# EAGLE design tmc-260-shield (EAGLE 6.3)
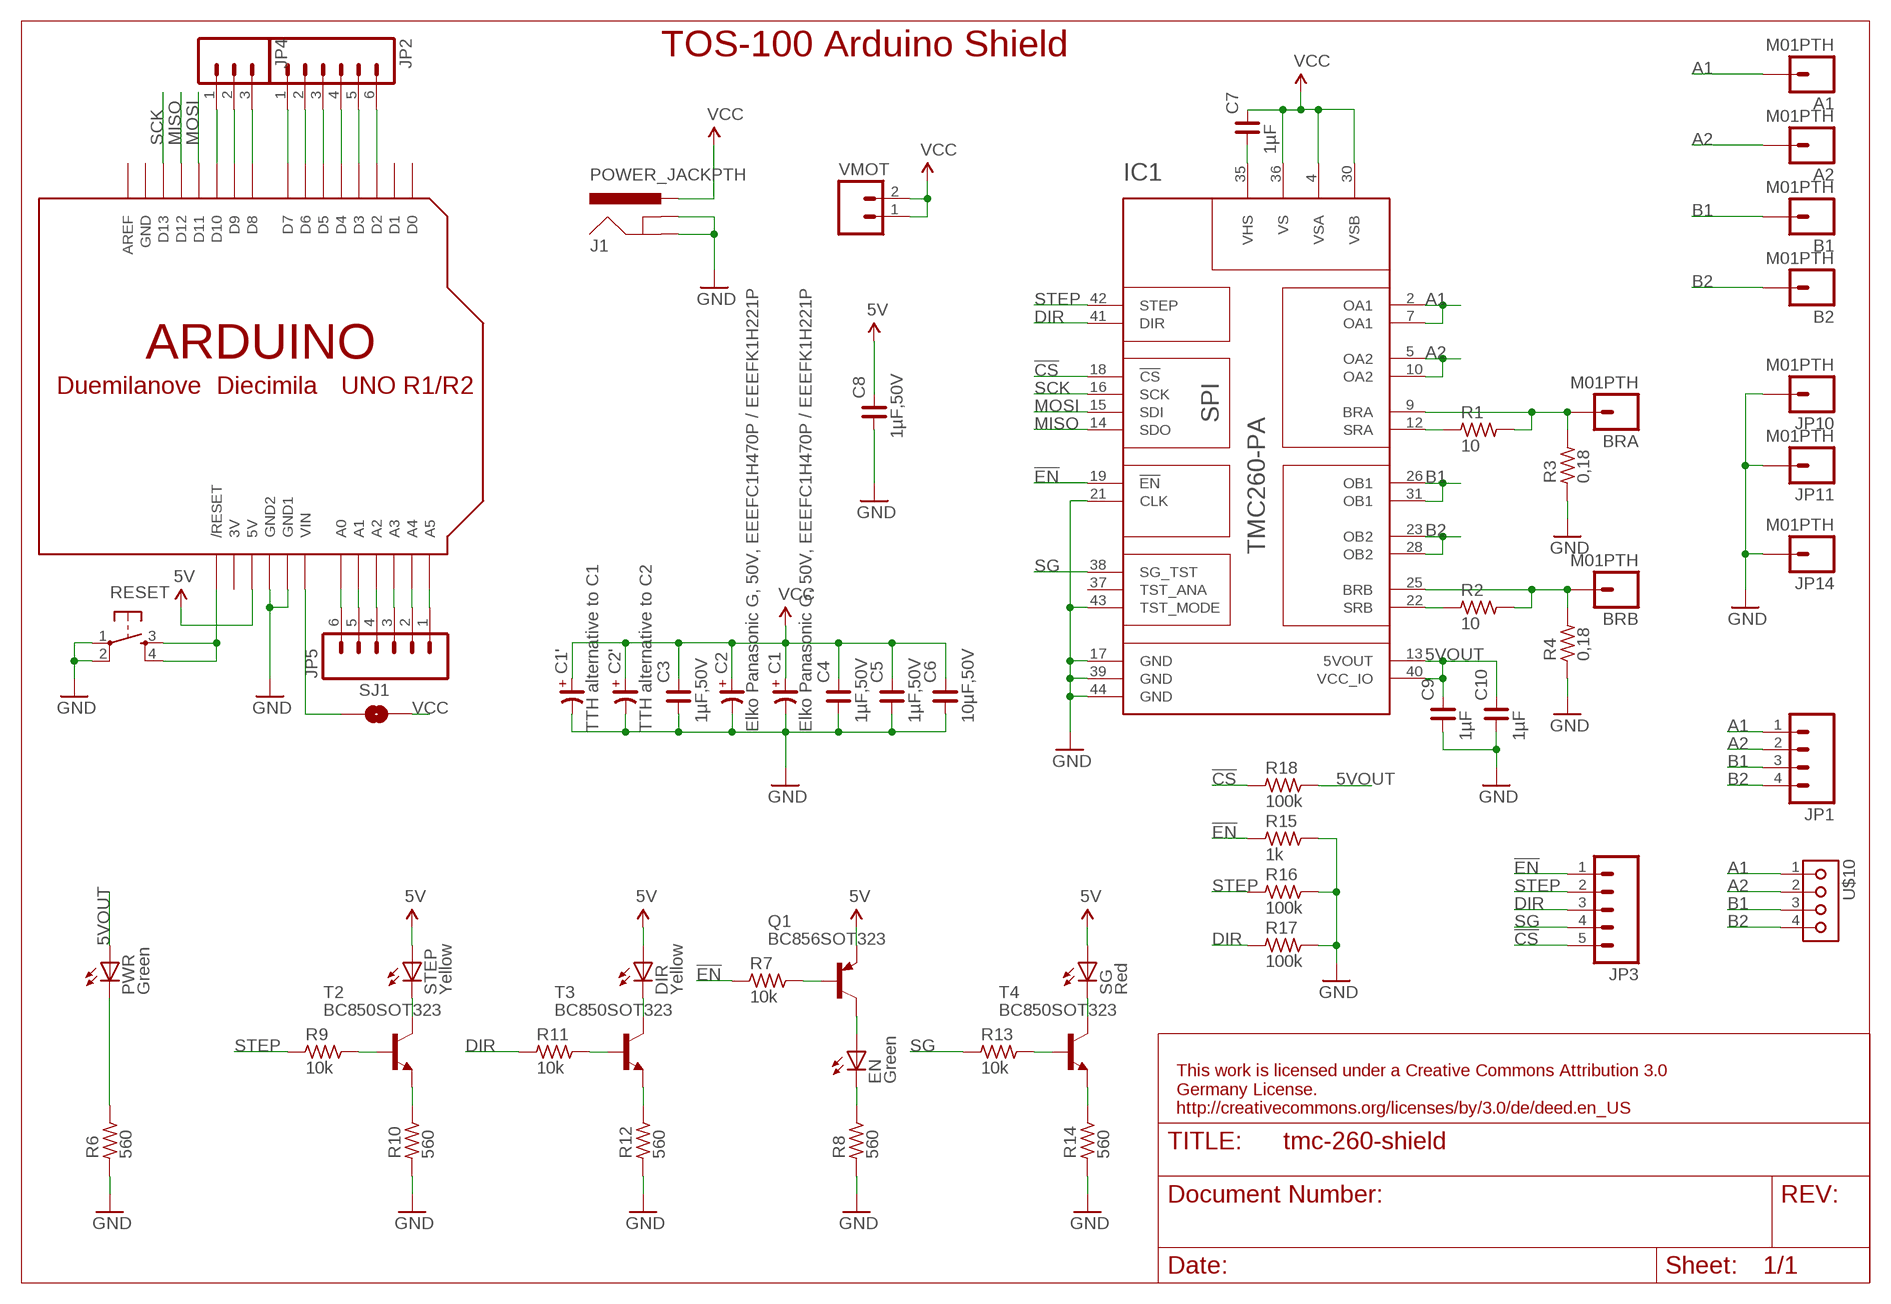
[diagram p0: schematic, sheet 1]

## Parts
A1  M01PTH  [1X01]
A2  M01PTH  [1X01]
B1  M01PTH  [1X01]
B2  M01PTH  [1X01]
BRA  M01PTH  [1X01]
BRB  M01PTH  [1X01]
C1  Elko Panasonic G, 50V, EEEFC1H470P / EEEFK1H221P  CP_SV-G  [CSV-G]
C1'  TTH alternative to C1  CP_E-035X100  [CE-035X100]
C2  Elko Panasonic G, 50V, EEEFC1H470P / EEEFK1H221P  CP_SV-G  [CSV-G]
C2'  TTH alternative to C2  CP_E-035X100  [CE-035X100]
C3  1µF,50V  C_0603  [C0603]
C4  1µF,50V  C_0603  [C0603]
C5  1µF,50V  C_0603  [C0603]
C6  10µF,50V  C_1206  [C1206]
C7  1µF  C_0603  [C0603]
C8  1µF,50V  C_0603  [C0603]
C9  1µF  C_0603  [C0603]
C10  1µF  C_0603  [C0603]
DIR  Yellow  LEDMICRO-SIDELED  [MICRO-SIDELED]
EN  Green  LEDMICRO-SIDELED  [MICRO-SIDELED]
IC1  TMC260-PA  [PQFP44_WITH_PADS]
J1  POWER_JACKPTH  [POWER_JACK_PTH]
JP1  M04SCREW  [SCREWTERMINAL-3.5MM-4]
JP2  M06SIP  [1X06]
JP3  M05PTH  [1X05]
JP4  M03PTH  [1X03]
JP5  M06SIP  [1X06]
JP10  M01PTH  [1X01]
JP11  M01PTH  [1X01]
JP14  M01PTH  [1X01]
PWR  Green  LEDMICRO-SIDELED  [MICRO-SIDELED]
Q1  BC856SOT323  BC858SOT323  [SOT323-BEC]
R1  10  R_0603  [R0603]
R2  10  R_0603  [R0603]
R3  0,18  R_2512  [R2512]
R4  0,18  R_2512  [R2512]
R6  560  R_0603  [R0603]
R7  10k  R_0603  [R0603]
R8  560  R_0603  [R0603]
R9  10k  R_0603  [R0603]
R10  560  R_0603  [R0603]
R11  10k  R_0603  [R0603]
R12  560  R_0603  [R0603]
R13  10k  R_0603  [R0603]
R14  560  R_0603  [R0603]
R15  1k  R_0603  [R0603]
R16  100k  R_0603  [R0603]
R17  100k  R_0603  [R0603]
R18  100k  R_0603  [R0603]
RESET  TAC_SWITCHSMD  [TACTILE_SWITCH_SMD]
SG  Red  LEDMICRO-SIDELED  [MICRO-SIDELED]
SJ1  SOLDERJUMPERNO  [SJ_2S-NO]
STEP  Yellow  LEDMICRO-SIDELED  [MICRO-SIDELED]
T2  BC850SOT323  [SOT323-BEC]
T3  BC850SOT323  [SOT323-BEC]
T4  BC850SOT323  [SOT323-BEC]
U$1  ARDUINOUNO  [ARDUINO]
U$10  KK4H  [KK-H-4]
VMOT  M021X02_NO_SILK  [1X02_NO_SILK]

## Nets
5V: C8.2 DIR.A Q1.E SG.A STEP.A U$1.5V
5VOUT: C9.2 C10.2 IC1.13(5VOUT) IC1.40(VCC_IO) PWR.A R18.2
!CS: IC1.18(!CS) JP3.5 R18.1
!EN: IC1.19(!EN) JP3.1 R7.1 R15.1
A1: A1.1 IC1.2(OA1) IC1.7(OA1) JP1.1 U$10.1
A2: A2.1 IC1.5(OA2) IC1.10(OA2) JP1.2 U$10.2
B1: B1.1 IC1.26(OB1) IC1.31(OB1) JP1.3 U$10.3
B2: B2.1 IC1.23(OB2) IC1.28(OB2) JP1.4 U$10.4
DIR: IC1.41(DIR) JP3.3 R11.1 R17.1
GND: C1'.- C1.- C2'.- C2.- C3.1 C4.1 C5.1 C6.1 C8.1 C9.1 C10.1 IC1.17(GND) IC1.21(CLK) IC1.39(GND) IC1.43(TST_MODE) IC1.44(GND) J1.GND J1.GNDBREAK JP10.1 JP11.1 JP14.1 R3.1 R4.1 R6.1 R8.1 R10.1 R12.1 R14.1 R15.2 R16.2 R17.2 RESET.1 RESET.2 U$1.GND1 U$1.GND2
MISO: IC1.14(SDO) U$1.D12
MOSI: IC1.15(SDI) U$1.D11
N$1: JP4.1 U$1.D10
N$2: JP4.2 U$1.D9
N$3: JP4.3 U$1.D8
N$4: JP2.1 U$1.D7
N$5: JP2.2 U$1.D6
N$6: JP2.3 U$1.D5
N$7: JP2.4 U$1.D4
N$8: JP2.5 U$1.D3
N$9: JP2.6 U$1.D2
N$10: JP5.1 U$1.A5
N$11: JP5.2 U$1.A4
N$12: JP5.3 U$1.A3
N$13: JP5.4 U$1.A2
N$14: JP5.5 U$1.A1
N$15: JP5.6 U$1.A0
N$16: R9.2 T2.B
N$17: RESET.3 RESET.4 U$1.RESET(/RESET)
N$18: SJ1.1 U$1.VIN
N$19: STEP.C T2.C
N$20: R10.2 T2.E
N$21: PWR.C R6.2
N$24: R11.2 T3.B
N$25: DIR.C T3.C
N$26: R12.2 T3.E
N$27: EN.A Q1.C
N$28: BRA.1 IC1.9(BRA) R1.2 R3.2
N$29: IC1.12(SRA) R1.1
N$30: BRB.1 IC1.25(BRB) R2.2 R4.2
N$31: IC1.22(SRB) R2.1
N$35: EN.C R8.2
N$36: Q1.B R7.2
N$38: R13.2 T4.B
N$39: SG.C T4.C
N$40: R14.2 T4.E
SCK: IC1.16(SCK) U$1.D13
SG: IC1.38(SG_TST) JP3.4 R13.1
STEP: IC1.42(STEP) JP3.2 R9.1 R16.1
VCC: C1'.+ C1.+ C2'.+ C2.+ C3.2 C4.2 C5.2 C6.2 C7.2 IC1.4(VSA) IC1.30(VSB) IC1.36(VS) J1.PWR SJ1.2 VMOT.1 VMOT.2
VHS: C7.1 IC1.35(VHS)
Unconnected: IC1.37(TST_ANA) U$1.AREF U$1.D0 U$1.D1

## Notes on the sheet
- TOS-100 Arduino Shield
- This work is licensed under a Creative Commons Attribution 3.0 
  Germany License.
  http://creativecommons.org/licenses/by/3.0/de/deed.en_US

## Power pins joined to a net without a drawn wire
3V: U$1.3V
GND: U$1.GND

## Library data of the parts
A1 A2 B1 B2 BRA BRB JP10 JP11 JP14 = SparkFun:M01: Header 1
C1 C1' C2 C2' = rc-master:CP_: POLARIZED CAP
C3-C10 = rc-master-smd:C_: NON-POLARIZED CAP
DIR EN PWR SG STEP = LED:LED: LED
IC1 = trinamic-2:TMC260-PA: TRINAMIC Energy Efficient Microstep Driver for up to 1.7A with coolStep&trade; Information given in this library is believed to be accurate and reliable. However no warranty is given for its correctness. Datasheet for TMC260/261/262 Description Energy Efficient Microstep Driver for up to 1.7A with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
J1 = SparkFun:POWER_JACK: Power Jack This is the standard 5.5mm barrel jack for power. The PTH is the most common, proven, reliable, footprint. All others are experimental. The Slot footprint only works if the mill layer is transmitted to the PCB fab house so be warned. Spark Fun Electronics SKU : PRT-00119. Mating wall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
JP1 = SparkFun:M04: Header 4 Standard 4-pin 0.1" header. Use with straight break away headers (SKU : PRT-00116), right angle break away headers (PRT-00553), swiss pins (PRT-00743), machine pins (PRT-00117), and female headers (PRT-00115). Molex polarized connector foot print use with SKU : PRT-08231 with associated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
JP2 JP5 = SparkFun:M06: Header 6 Standard 6-pin 0.1" header. Use with straight break away headers (SKU : PRT-00116), right angle break away headers (PRT-00553), swiss pins (PRT-00743), machine pins (PRT-00117), and female headers (PRT-00115). Molex polarized connector foot print use with SKU : PRT-08094 with associated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
JP3 = SparkFun:M05: Header 5 Standard 5-pin 0.1" header. Use with straight break away headers (SKU : PRT-00116), right angle break away headers (PRT-00553), swiss pins (PRT-00743), machine pins (PRT-00117), and female headers (PRT-00115). Molex polarized connector foot print use with SKU : PRT-08230 with associated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
JP4 = SparkFun:M03: Header 3 Standard 3-pin 0.1" header. Use with straight break away headers (SKU : PRT-00116), right angle break away headers (PRT-00553), swiss pins (PRT-00743), machine pins (PRT-00117), and female headers (PRT-00115). Molex polarized connector foot print use with SKU : PRT-08232 with associated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
Q1 = additional:BC858*: PNP Transistror
R1-R4 R6-R18 = rc-master-smd:R_: RESISTOR
RESET = SparkFun:TAC_SWITCH: Momentary Switch Button commonly used for reset or general input. Spark Fun Electronics SKU : COM-00097
SJ1 = SparkFun:SOLDERJUMPER: Solder Jumper
T2-T4 = additional:BC850: NPN TRANSISTOR
U$1 = adafruit:ARDUINO: Arduino Diecimila/Duemilanove Make a shield with ease, this package has all the named pins as well as the two mounting drill holes and an outline of the USB and DC power connector. The outline is on the DIMENSION layer, so if your board house uses it they will cut the outline to match.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
U$10 = molex-kk:KK4*
VMOT = SparkFun:M02: Header 2

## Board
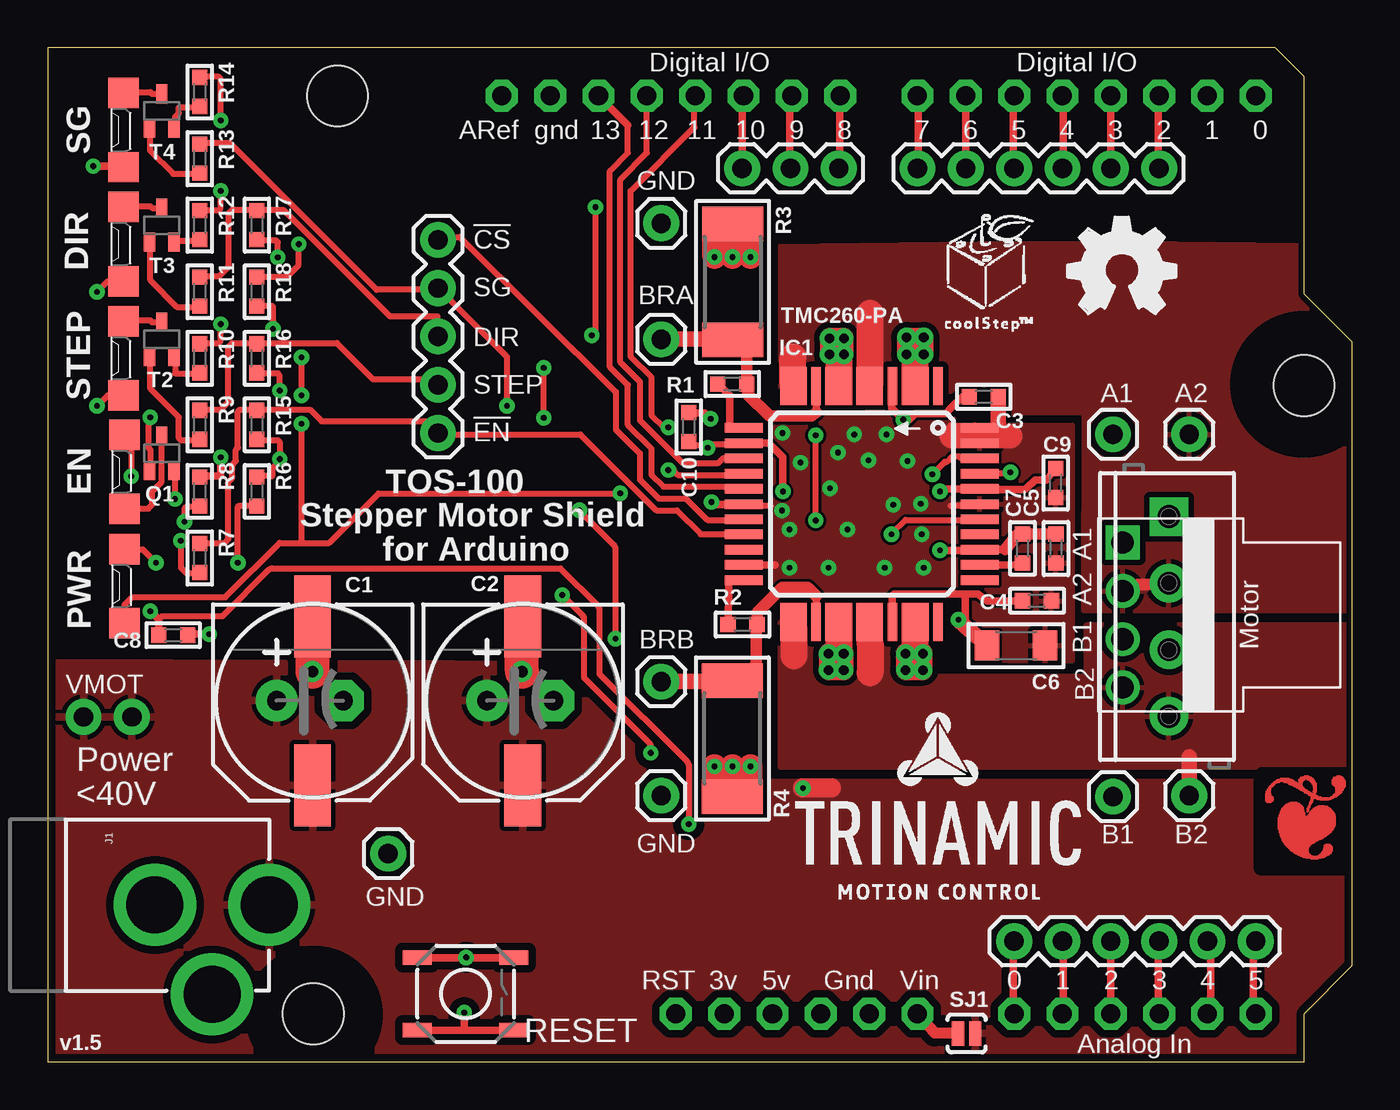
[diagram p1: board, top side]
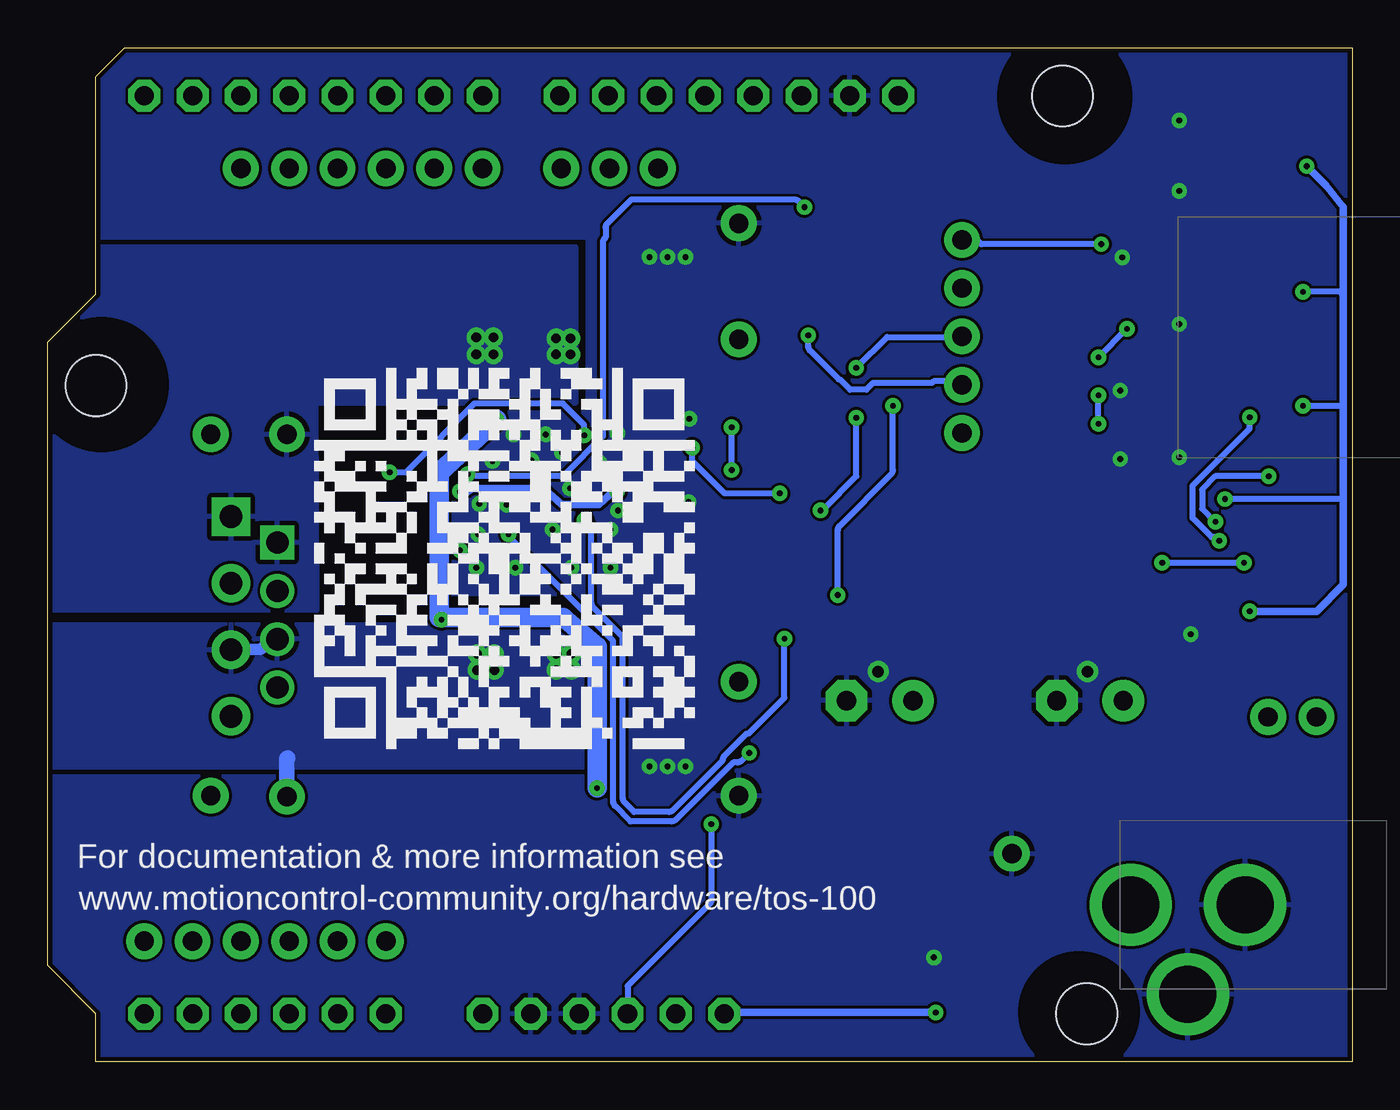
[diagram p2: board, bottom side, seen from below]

Size 68.58 x 53.34 mm. Coordinates in mm from the lower left corner, seen from the top.
Copper layers (1*16): Top 0.035mm / dielectric 1.5mm / Bottom 0.035mm
Design rules "eurocircuits-PCB-Proto": minimum track width 0.15mm, minimum drill 0.25mm, track to track 0.15mm, track to pad 0.15mm, pad to pad 0.15mm, via to via 0.15mm, smd to smd 0.15mm, copper to edge 10mil, drill to drill 8mil, minimum pad ring 12mil, minimum via ring 10mil, stop-mask expansion 4mil, vias tented up to drill 25mil, thermal gap 10mil
tRestrict: area 62.9,32.5 to 69.1,38.8; area 10.8,-0.7 to 17.2,5.7; 4 lines
bRestrict: area 62.6,32.5 to 68.9,38.8; area 12,47.6 to 18.3,53.9; area 11.2,-0.6 to 17.6,5.8

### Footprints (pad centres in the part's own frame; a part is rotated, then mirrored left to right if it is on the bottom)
1X01 = drill 1.016 pad 1.88: 1 0,0
CSV-G = smd 4.318 x 1.93: + -4.445,0; - 4.445,0
CE-035X100 = drill 1.016 pad 2.184: + -1.905,0 | drill 1.016 pad 2.184 octagon: - 1.587,0
C0603 = smd 0.8 x 0.8: 1 -0.762,0; 2 0.762,0
C1206 = smd 1.3 x 1.6: 1 -1.524,0; 2 1.524,0
MICRO-SIDELED = smd 1.6 x 1.6: A 0,1.95; C 0,-1.95
PQFP44_WITH_PADS = smd 2 x 0.5: 1 -6.327,4.254; 4 -6.327,1.854; 9 -6.327,-2.146; 25 6.073,-2.146; 30 6.073,1.854; 33 6.073,4.254 | smd 2 x 1.4: 2 -6.327,3.06; 5 -6.327,0.66; 7 -6.327,-0.965; 10 -6.327,-3.34; 23 6.073,-3.34; 26 6.073,-0.965; 28 6.073,0.66; 31 6.073,3.06 | smd 0.5 x 2: 12 -4.127,-5.946; 13 -3.327,-5.946; 14 -2.527,-5.946; 15 -1.727,-5.946; 16 -0.927,-5.946; 17 -0.127,-5.946; 18 0.673,-5.946; 19 1.473,-5.946; 20 2.273,-5.946; 21 3.073,-5.946; 22 3.873,-5.946; 34 3.873,6.454; 35 3.073,6.454; 36 2.273,6.454; 37 1.473,6.454; 38 0.673,6.454; 39 -0.127,6.454; 40 -0.927,6.454; 41 -1.727,6.454; 42 -2.527,6.454; 43 -3.327,6.454; 44 -4.127,6.454
POWER_JACK_PTH = drill 2.997 pad 4.318: GND 0,7.7; GNDBREAK 4.7,10.7; PWR 0,13.7
SCREWTERMINAL-3.5MM-4 = drill 1.2 pad 2.032 square: 1 0,0 | drill 1.2 pad 2.032: 2 3.5,0; 3 7,0; 4 10.5,0
1X06 = drill 1.016 pad 1.88: 1 0,0; 2 2.54,0; 3 5.08,0; 4 7.62,0; 5 10.16,0; 6 12.7,0
1X05 = drill 1.016 pad 1.88: 1 0,0; 2 2.54,0; 3 5.08,0; 4 7.62,0; 5 10.16,0
1X03 = drill 1.016 pad 1.88: 1 0,0; 2 2.54,0; 3 5.08,0
SOT323-BEC = smd 0.6 x 1: B -0.65,-0.9; C 0,0.9; E 0.65,-0.9
R0603 = smd 0.8 x 0.8: 1 -0.762,0; 2 0.762,0
R2512 = smd 1.8 x 3.2: 1 -3.048,0; 2 3.048,0
TACTILE_SWITCH_SMD = smd 1.524 x 0.762: 1 -2.54,1.905; 2 2.54,1.905; 3 -2.54,-1.905; 4 2.54,-1.905
SJ_2S-NO = smd 0.635 x 1.27: 1 -0.45,0; 2 0.45,0
ARDUINO = drill 1 pad 1.676 octagon: 3V 35.56,2.54; 5V 38.1,2.54; A0 50.8,2.54; A1 53.34,2.54; A2 55.88,2.54; A3 58.42,2.54; A4 60.96,2.54; A5 63.5,2.54; AREF 23.876,50.8; D0 63.5,50.8; D1 60.96,50.8; D2 58.42,50.8; D3 55.88,50.8; D4 53.34,50.8; D5 50.8,50.8; D6 48.26,50.8; D7 45.72,50.8; D8 41.656,50.8; D9 39.116,50.8; D10 36.576,50.8; D11 34.036,50.8; D12 31.496,50.8; D13 28.956,50.8; GND 26.416,50.8; GND1 43.18,2.54; GND2 40.64,2.54; RESET 33.02,2.54; VIN 45.72,2.54 | hole 3.2: 15.24,50.8; 66.04,35.56; 13.97,2.54
KK-H-4 = drill 1.168 square: 1 0,3.81 | drill 1.168: 2 0,1.27; 3 0,-1.27; 4 0,-3.81
1X02_NO_SILK = drill 1.016 pad 1.88: 1 0,0; 2 2.54,0

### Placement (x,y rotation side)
A1  56,33 0 top
A2  60,33 0 top
B1  56,13.95 0 top
B2  60,14 0 top
BRA  32.25,38 0 top
BRB  32.25,20 0 top
C1  13.93,18.98 90 top
C1'  25,19 0 top
C2  24.98,18.98 90 top
C2'  13.95,19 0 top
C3  49.2,34.98 180 top
C4  52,24.25 180 top
C5  53,27 90 top
C6  50.9,21.9 180 top
C7  51.24,27 90 top
C8  6.6,22.45 180 top
C9  52.98,30.44 90 top
C10  33.7,33.38 270 top
DIR  4,43 180 top
EN  4.04,31.03 180 top
IC1  42.55,29.21 270 top
J1  -2.06,8.26 270 top
JP1  58.94,28.68 270 top
JP2  45.72,46.99 0 top
JP3  20.52,33.07 90 top
JP4  36.51,46.99 0 top
JP5  63.5,6.35 180 top
JP10  32.25,14 0 top
JP11  32.25,44.1 0 top
JP14  17.9,10.95 0 top
PWR  4.04,25.02 180 top
Q1  6,32 0 top
R1  35.98,35.65 0 top
R2  36.52,23 0 top
R3  36.01,41.02 270 top
R4  35.99,17 90 top
R6  11,30 270 top
R7  8,26.5 270 top
R8  8,30 270 top
R9  8,33.5 270 top
R10  8,37 270 top
R11  8,40.5 270 top
R12  8,44 270 top
R13  8,47.5 270 top
R14  8,51 270 top
R15  11,33.5 270 top
R16  11,37 270 top
R17  11,44 270 top
R18  11,40.5 270 top
RESET  21.97,3.58 0 top
SG  4,49 180 top
SJ1  48.3,1.5 0 top
STEP  4,37 180 top
T2  6,38 0 top
T3  6,44 0 top
T4  6,50 0 top
U$1  0,0 0 top
U$5  [LOGO]  39.3,8.55 0 top
U$9  [COOLSTEP]  46.85,38.25 0 top
U$10  56.5,23.5 0 top
U$11  [OSHW_FILLX200_NOTEXT]  53.62,39.35 0 top
U$12  [SMALL_LOGO_COPPER]  63.5,10.3 0 top
U$13  [QR-TMC-100-BOTTOM-BIG]  34.6,16.5 0 top
VMOT  1.89,18.14 0 top

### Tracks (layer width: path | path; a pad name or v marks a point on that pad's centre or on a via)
5V  (via drill 0.3)
  Top 0.305: 4,41.1 DIR.A 3.15,41.05 v2.6,40.5 | 4,35.1 STEP.A 3.15,35.05 v2.6,34.5 | v6.7,29.6 6.7,31.1 Q1.E | 5.84,23.26 6.03,23.45 9.2,23.45 11.61,25.86 arc-45 11.83,25.95 26.95,25.95 28.91,23.99 arc-45 29,23.77 29,20.4 33.61,15.79 arc-45 33.7,15.57 v33.7,12.5
  Top 0.406: v2.4,47.1 4,47.1 SG.A | C8.2 5.84,23.26 v5.4,23.7
  Bottom 0.305: 0.47,29.6 v6.7,29.6 | v2.6,40.5 0.67,40.5 0.47,40.3 | v2.6,34.5 0.57,34.5 0.47,34.4 | v33.7,12.5 33.7,8.4 38.1,4 U$1.5V
  Bottom 0.406: v2.4,47.1 1.4,46.1 0.47,44.96 0.47,40.3 0.47,34.4 0.47,29.6 0.47,25.1 1.87,23.7 v5.4,23.7
5VOUT  (via drill 0.3)
  Top 0.305: C10.2 33.7,32.4 34.7,32.4 v34.7,32.3 34.8,32.5 36.4,32.5 IC1.13 | 13.35,27.3 14.8,27.3 17.4,29.9 v30.1,29.9 | v11.85,38.55 11.85,39.7 11.8,39.75 R18.2 | v13.35,35.05 v13.35,37.05 | 13.35,27.3 v13.35,33.55 | 13.35,27.3 12.2,27.3 9.35,24.45 4.45,24.45 4.05,24.05 PWR.A
  Top 0.406: IC1.40 49,30.12 | 36.75,32.5 IC1.13 36.61,32.55 37.9,32.55 38.65,31.8 v38.65,30 | IC1.40 48.88,30.12 47.02,30.12 v46.9,30 | IC1.40 49.2,30.1 51.35,30.1 51.5,30.2 51.9,30.6 52.5,30.6 C9.2
  Bottom 0.305: v30.1,29.9 33,29.9 34.7,31.6 v34.7,32.3 | v13.35,37.05 v11.85,38.55 | v13.35,33.55 v13.35,35.05
  Bottom 0.406: v46.9,30 46.5,30 46.25,30.15 42.5,30.15 41.55,29.3 39.6,29.3 38.85,30 v38.65,30
!CS  (via drill 0.3)
  Top 0.305: IC1.18 36.5,28.5 34.67,28.5 33.55,29.62 32.12,29.62 31.12,30.62 31.12,32 29.88,33.25 29.88,35.23 21.68,43.38 20.75,43.38 20.62,43.25 JP3.5 | R18.1 11,41.3 12.6,41.3 13.2,41.9 v13.2,43
  Bottom 0.305: v13.2,43 19.5,43 19.7,43.2 20.5,43.2 JP3.5
!EN
  Top 0.305: IC1.19 36.5,27.75 34.33,27.75 33.08,29 32,29 28,33 20.62,33 JP3.1 20.5,33.2 20.5,33.7 14.4,33.7 13.8,34.3 11.1,34.3 R15.1 10.9,34.3 10.1,34.3 10,34.2 10,32.3 9.9,32.2 9.9,31.6 9.7,31.4 9.7,30.7 9.5,30.5 9.5,27.5 9.3,27.3 8,27.3 R7.1
A1  (via drill 0.5)
  Top 0.813: IC1.2 45.6,35.75 | IC1.7 41.6,35.75
  Top 1.016: 41.6,37.55 v41.1,38.05 v41.1,37.2 v41.85,37.2 41.85,38.1 41.1,38.1 | 45.6,37.75 v45.15,38.1 | v45.15,38.1 v46.05,38.1 v46.05,37.2 | v45.15,38.1 v45.15,37.2
  Top 1.422: 41.6,35.75 41.6,37.55 | 45.6,35.75 45.6,37.75
  other vias: 41.85,38.05
  pour Bottom: 70.5,42.88 40.83,42.88 40.83,34.62 54.48,34.62 54.42,23.75 70.5,23.75
A2
  Top 0.61: 56.3,24.7 57.3,25.1 58.8,25.1
  Top 0.813: IC1.5 43.23,35.67 | IC1.10 39.17,35.65
  Top 1.422: 43.23,35.67 43.23,39.38 | 39.17,35.65 39.17,37.08
  pour Top (isolate 0.305): 38.5,34.85 48.15,35.05 48.15,34.15 54.45,34.15 54.42,23.75 69.12,23.75 69.75,42.88 arc2 38.5,42.88
B1  (via drill 0.5)
  Top 0.305: v41.84,21.46 41.83,21.35
  Top 0.813: 41.7,22.6 41.62,22.62 41.58,22.86 IC1.26
  Top 1.016: 41.7,22.6 41.7,22.5 41.6,22.8 | 41.85,21.5 41.6,21.1 | 41.85,21.5 v41.85,20.6 v41.05,20.6 41.05,21.5 | 41.83,21.35 41.85,21.5 | 45.6,21 45.49,21 v45.1,20.61 | v45.1,20.6 v46,20.6 46,21.5 45.1,21.5 v45.1,21.46 v45.1,20.6
  Top 1.422: 41.6,21.1 41.6,22.8 | 45.6,21 IC1.31
  Bottom 0.61: 56.6,22.3 57.4,21.7 58.8,21.7
  Bottom 0.813: B1.1 56,15.95 55.95,16
  other vias: 41.05,21.46 46,21.46
  pour Bottom: 40.45,15.5 69.25,15.5 69.25,23 41.75,23 40.4,21.93 40.4,21.1
B2
  Top 0.813: 43.23,22.01 IC1.28 | 39.23,22.75 IC1.23 | U$10.4 56.5,19.62 | B2.1 60,16.05
  Top 1.422: 43.23,22.01 43.23,20.47 | 39.23,22.75 39.23,21.38
  pour Top (isolate 0.305): 38.5,23.12 46.4,22.9 46.4,20.3 54.6,20.3 54.6,23 69,23 69.12,15.5 38.5,15.5 arc1
DIR  (via drill 0.3)
  Top 0.305: v26.07,33.88 v26.07,36.5 | v40.38,28.48 v40.38,32.95 | 49,30.88 IC1.41 50.39,30.94 v50.6,31 | R11.1 8,41.3 9,41.3 9.5,41.8 9.5,44.6 9.7,44.8 11,44.8 R17.1 11.1,44.8 12.4,44.8 18,39.2 20.5,39.2 20.5,38.2 JP3.3 | v29.85,22.25 29.85,26.97 arc45 29.76,27.19 v27.95,29
  Bottom 0.305: v26.07,33.88 26.07,30.8 27.82,29.05 arc45 v27.95,29 | v26.07,36.5 24.45,38.12 20.62,38.12 JP3.3 | v40.38,28.48 40,28.25 40,24.13 arc-45 39.91,23.91 38.35,22.35 38.35,13.88 arc-45 38.26,13.66 37.75,13.15 35.93,13.15 arc-45 35.71,13.24 33.1,15.85 33.1,15.87 arc45 33.01,16.09 31.85,17.25 arc-45 31.68,17.32 29.85,19.15 v29.85,22.25 | v40.38,32.95 40.38,33.5 41.5,34.62 46.15,34.62 47.8,32.98 47.9,32.85 49.75,31 v50.6,31
GND  (via drill 0.3, 0.6)
  Top 0.254: 36,43.87 36.01,43.87 R3.1 | v35.05,15.54 35,15.5 35.05,15.5
  Top 0.305: 47.45,29.25 48.75,29.25 IC1.39 | 47.45,32.5 48.75,32.5 IC1.43 | 47.45,33.48 48.75,33.48 IC1.44 | 38.02,29.25 36.73,29.25 IC1.17 | v9.1,49.5 9.1,51.7 9,51.8 8,51.8 R14.1 | v9.1,45.8 9.1,44.9 9,44.8 8,44.8 R12.1 | v12.1,42.3 12.1,43.1 12,43.2 11,43.2 R17.2 | v9.1,38.8 9.1,37.9 9,37.8 8,37.8 R10.1 | v12.2,35.3 12.2,36.1 12.1,36.2 11,36.2 R16.2 | R15.2 11,32.7 12.1,32.7 12.2,32.6 v12.2,31.7 12.1,31.6 12.1,31.5 11.8,31.2 11.8,30.8 11,30.8 R6.1
  Top 0.406: C10.1 33.75,34.12 34.55,34.12 v34.85,33.83 | IC1.21 38.25,26.14 38.25,26.12 | v9.1,31.8 9.1,30.9 9,30.8 8,30.8 R8.1 | RESET.1 21.98,5.49 v22,5.5 22.02,5.49 RESET.2 | C8.1 7.47,22.5 v8.5,22.5 | 36.5,29.3 35.23,29.3 arc-45 35.01,29.39 34.9,29.5 arc45 34.9,29.49 v34.9,29.45
  Top 0.813: C3.1 49.96,33.19 50.25,32.9
  Top 1.27: R4.1 v35.99,15.54 | v36,42.33 36,43.87 | v35.05,42.33 35.05,43.87 | v36.95,42.33 36.95,43.87 | 35.05,13.96 35.05,15.5 v35.05,15.54 | 36.95,13.96 v36.95,15.54 | 47.5,32.9 50.25,32.9 50.6,32.9
  Top 1.778: v13.93,20.53 C1.- | v24.93,20.53 C2.-
  other vias: 38.62,33.07 39.57,31.52 38.59,29 45.9,29.34 38.99,26 41.05,26 43.99,26 45.95,27.75 46.05,26 44.45,29.3 45.2,31.59 44.09,32.99 43.15,31.64 42.4,32.99 41.55,32.05 41.12,30.17 38.99,28 42.05,28
  pour Bottom: 70.48,-1.91 -1.27,-1.91 -1.27,54.61 66.75,54.73 66.62,43.38 40.2,43.38 40.2,34.12 47.38,34.12 47.38,24.62 41.5,24.6 41.5,23.82 39.52,22.23 39.52,15 70.25,15 70.25,10
  pour Top: 38.02,25.02 38.02,33.8 38.35,34.12 47.52,34.23 47.65,33.5 53.85,33.5 53.85,21.05 47.1,21.1 47.1,23.9 46.75,24.23 46.83,24.8 38.35,24.7
MISO
  Top 0.305: 36.5,31.75 35.5,31.75 35.25,31.5 33.38,31.5 31.12,33.75 31.12,35.77 30.1,36.8 30.1,46.4 31.5,47.8 U$1.D12
  Top 0.406: 36.5,31.75 IC1.14 | 31.12,50.5 31.38,50.75 U$1.D12
MOSI  (via drill 0.3)
  Top 0.305: 32.38,33.38 31.75,34 31.75,36 30.65,37.1 30.65,45.8 34,49.15 34,50.76 U$1.D11 | 32.88,31.12 33.12,30.88 36.5,30.88 IC1.15
  Top 0.406: v32.62,33.38 32.38,33.38 | v32.62,31.12 32.88,31.12 | U$1.D11 34,50.75
  Bottom 0.305: v32.62,31.12 v32.62,33.38
N$1
  Top 0.406: JP4.1 36.5,50.75 U$1.D10
N$2
  Top 0.406: JP4.2 39,47 39,50.75 U$1.D9
N$3
  Top 0.406: JP4.3 41.62,47 41.62,50.75 U$1.D8
N$4
  Top 0.406: JP2.1 45.75,47 45.75,50.75 U$1.D7
N$5
  Top 0.406: JP2.2 48.25,50.75 U$1.D6
N$6
  Top 0.406: JP2.3 50.75,47 50.75,50.75 U$1.D5
N$7
  Top 0.406: JP2.4 53.38,47 53.38,50.75 U$1.D4
N$8
  Top 0.406: JP2.5 55.88,50.75 U$1.D3
N$9
  Top 0.406: JP2.6 58.38,47 58.38,50.75 U$1.D2
N$10
  Top 0.406: U$1.A5 63.5,2.62 63.38,2.75 63.38,6.12 63.5,6.25 JP5.1
N$11
  Top 0.406: U$1.A4 61,2.62 61.12,2.75 61.12,6.12 61,6.25 JP5.2
N$12
  Top 0.406: U$1.A3 58.38,2.62 58.38,6.25 JP5.3
N$13
  Top 0.406: U$1.A2 55.88,2.62 55.88,6.25 JP5.4
N$14
  Top 0.406: JP5.5 53.38,6.25 53.38,2.62 U$1.A1
N$15
  Top 0.406: JP5.6 50.75,6.25 50.75,2.62 U$1.A0
N$16
  Top 0.305: R9.2 8,32.7 7,32.7 6.9,32.8 6.9,33.9 5.4,35.4 5.4,37.1 T2.B
N$17  (via drill 0.3)
  Top 0.406: RESET.3 21.9,1.68 | 21.9,1.68 RESET.4 | 21.9,1.68 v21.9,2.6
  Bottom 0.406: v21.9,2.6 32.96,2.6 U$1.RESET
N$18
  Top 0.61: U$1.VIN 46.62,1.53 SJ1.1
N$19
  Top 0.305: T2.C 5.5,38.9 5.4,39 4,39 STEP.C
N$20
  Top 0.305: R10.2 8,36.2 6.7,36.2 6.7,37.1 T2.E
N$21  (via drill 0.3)
  Top 0.305: v5.7,26.25 5,26.95 4.05,26.95 PWR.C | v10,26.25 10,29.2 10.05,29.25 R6.2
  Bottom 0.305: v5.7,26.25 v10,26.25
N$24
  Top 0.305: R11.2 8,39.7 6.8,39.7 5.4,41.1 5.4,43.1 T3.B
N$25
  Top 0.305: T3.C 5.5,44.9 5.4,45 4,45 DIR.C
N$26
  Top 0.305: R12.2 8,43.2 6.7,43.2 6.7,43.1 T3.E
N$27
  Top 0.305: Q1.C 6,30.5 5.5,30 5.5,29.3 5.3,29.1 4.1,29.1 EN.A
N$28
  Top 0.406: IC1.9 40.4,34.15 40.4,34.1
  Top 0.61: 40.4,34.15 40.15,33.95 37.95,33.95 36.8,35.1 36.8,35.65 R1.2 36.75,35.95 36.75,37.9 36.7,37.95 36.05,37.95 R3.2
  Top 0.813: BRA.1 35.98,38 R3.2
N$29
  Top 0.406: 36.5,33.38 IC1.12 36.54,33.4 35.9,33.4 35.85,33.6 35.85,35.05 35.25,35.65 R1.1
N$30
  Top 0.406: 40.4,24.5 IC1.25
  Top 0.61: 40.4,24.5 39.95,24.95 38.6,24.95 37.29,23.64 R2.2 37.25,23.02 37.25,20.9 36.4,20.05 R4.2
  Top 0.813: BRB.1 35.94,20 R4.2
N$31
  Top 0.406: R2.1 35.81,24.91 35.8,25.4 36.54,25.4 IC1.22
N$35  (via drill 0.3)
  Top 0.305: R8.2 8,29.2 7.3,29.2 7.2,29.1 v7.2,28.4 7.2,28.3 | v4.4,30.8 4.4,33 4.1,33 EN.C
  Bottom 0.305: v7.2,28.4 7.9,29.1 7.9,30.1 7.2,30.8 v4.4,30.8
N$36  (via drill 0.3)
  Top 0.305: R7.2 8,25.7 7.3,25.7 7,26 v7,27.4 | v5.4,33.9 5.4,33.6 5.3,33.5 5.3,32.3 5.4,32.2 5.4,31.1 Q1.B
  Bottom 0.305: v7,27.4 7.2,27.6 7.4,27.6 8.4,28.6 8.4,30.3 5.4,33.3 v5.4,33.9
N$38
  Top 0.305: R13.2 8,46.7 6.6,46.7 5.4,47.9 5.4,49.1 T4.B
N$39
  Top 0.305: T4.C 5.5,50.9 5.4,51 4,51 SG.C
N$40
  Top 0.305: R14.2 8,50.2 6.9,50.2 6.9,49.9 6.7,49.7 6.7,49.1 T4.E
SCK
  Top 0.305: 36.5,30.12 35.88,30.12 35.75,30.25 32.38,30.25 31.75,30.88 31.75,32.25 30.5,33.5 30.5,35.6 29.55,36.55 29.55,46.85 30.5,47.8 30.5,49.25
  Top 0.406: 36.5,30.12 IC1.16 | 30.5,49.25 29,50.75 U$1.D13
SG  (via drill 0.3)
  Top 0.305: v44.35,27.75 45.1,28.5 48.88,28.5 IC1.38 | 20.4,40.6 17.3,40.6 9.6,48.3 8,48.3 R13.1 | v24.15,34.5 24.15,37.06 JP3.4 | v31.7,16.25 31.7,16.57 arc45 31.61,16.79 28.2,20.2 28.2,23.27 arc45 28.11,23.49 v27.05,24.55
  Top 0.406: JP3.4 20.4,40.6
  Bottom 0.305: v44.35,27.75 arc-45 44.28,27.58 38.85,22.15 38.85,13.68 arc-45 38.76,13.46 37.95,12.65 35.78,12.65 arc-45 35.56,12.74 32.55,15.75 32.33,15.75 arc-45 32.11,15.84 v31.7,16.25 | v27.05,24.55 27.05,27.97 arc45 26.96,28.19 24.24,30.91 arc-45 24.15,31.13 v24.15,34.5
STEP  (via drill 0.3)
  Top 0.305: IC1.42 48.85,31.75 48,31.75 47.9,31.85 47.55,31.85 47.25,31.55 47.15,31.55 v46.5,30.9 | R9.1 8,34.3 9.1,34.3 9.5,34.7 9.5,37.6 9.7,37.8 11,37.8 R16.1 11.1,37.8 15.2,37.8 17.1,35.9 20.5,35.9 20.5,35.7 JP3.2 | v28.8,44.95 28.8,38.53 arc-45 28.71,38.31 v28.6,38.2
  Bottom 0.305: v46.5,30.9 46.4,30.8 41.63,30.8 arc-45 41.41,30.89 39.4,32.9 39.4,43.07 arc45 39.31,43.29 39.25,43.35 39.25,43.87 arc45 39.16,44.09 37.9,45.35 29.33,45.35 arc45 29.11,45.26 v28.8,44.95 | JP3.2 20.55,35.6 21.15,35.6 21.35,35.8 22,35.8 22.1,35.7 25.2,35.7 25.55,35.35 26.4,35.35 26.95,35.9 27,35.9 28.51,37.41 arc45 28.6,37.63 v28.6,38.2
VCC  (via drill 0.3)
  Top 0.406: IC1.4 44.38,35.5 44.38,34.38 v44.98,33.77 45.27,33.77 45.6,34.1 47.2,34.1 47.5,34.4 48.1,34.99 C3.2 | IC1.36 49,26.88 | 44.38,23.12 IC1.30 44.4,23.2 44.4,24.5 44.5,24.6 48.24,24.6 | IC1.36 50.34,26.94 | 50.95,27.7 51.52,27.7 C7.2 | C5.2 | IC1.36 48.8,26.9 v46.9,26.9 46.8,26.9 | v47.88,23.25 48.24,23.25 48.24,24.6 | C4.2 49.4,24.25 48.9,24.6 48.24,24.6
  Top 0.61: 50.34,26.94 50.95,27.7 | C7.2 C5.2
  Top 0.813: C6.2 48.23,22.9 v47.88,23.25
  Top 1.016: v39.7,14.4 41.2,14.4
  Bottom 0.305: v44.98,33.77 44.75,33.75
  Bottom 0.406: 48,23.38 v47.88,23.25 | 48,26.9 v46.9,26.9
  Bottom 1.016: v44.98,33.77 48,31 48,26.9 48,23.38 41.48,23.38 39.7,21.85 v39.7,14.4
  pour Top (isolate 0.406): -0.85,21 28.85,20.9 33.5,14.7 69.65,14.7 69.75,-0.88 -0.75,-0.88
VHS
  Top 0.406: 49,26.12 IC1.35 50.66,26.14 50.9,26.15 51.25,26.15 C7.1

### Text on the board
tNames: GND | !CS | SG | DIR | STEP | !EN | TOS-100 | Stepper Motor Shield | for Arduino | A1 | A2 | B1 | Motor | B2 | Power | <40V | GND | GND | v1.5 | This work is licensed under a / Creative Commons Attribution 3.0 Germany License.
bNames: For documentation & more information see | www.motioncontrol-community.org/hardware/tos-100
